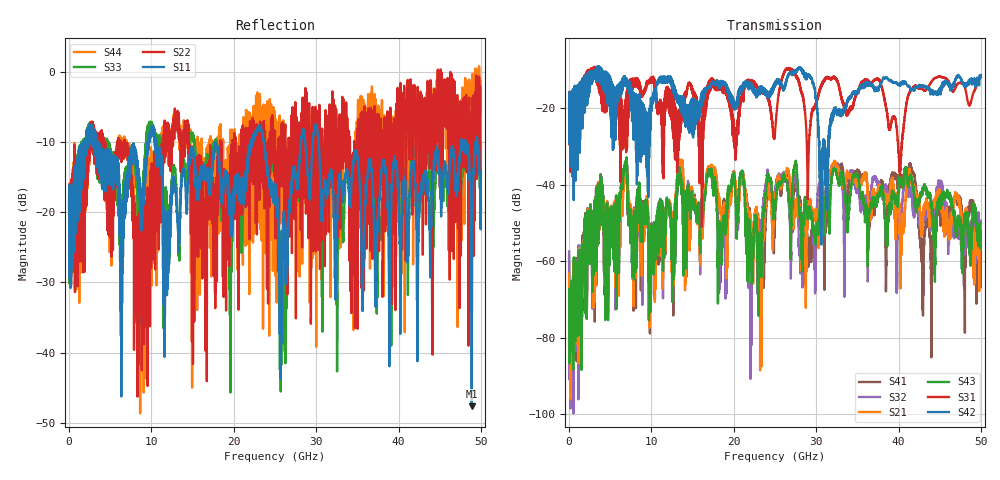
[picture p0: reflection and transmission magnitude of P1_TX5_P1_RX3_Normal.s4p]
!Keysight Technologies,N5225B,MY57041031,A.13.20.10
!Date: Friday, May 31, 2019 11:17:32
!Correction: S11(Full 4 Port(1,2,3,4))
!S12(Full 4 Port(1,2,3,4))
!S13(Full 4 Port(1,2,3,4))
!S14(Full 4 Port(1,2,3,4))
!S21(Full 4 Port(1,2,3,4))
!S22(Full 4 Port(1,2,3,4))
!S23(Full 4 Port(1,2,3,4))
!S24(Full 4 Port(1,2,3,4))
!S31(Full 4 Port(1,2,3,4))
!S32(Full 4 Port(1,2,3,4))
!S33(Full 4 Port(1,2,3,4))
!S34(Full 4 Port(1,2,3,4))
!S41(Full 4 Port(1,2,3,4))
!S42(Full 4 Port(1,2,3,4))
!S43(Full 4 Port(1,2,3,4))
!S44(Full 4 Port(1,2,3,4))
!S4P File: Measurements: <S11,S12,S13,S14>,
!<S21,S22,S23,S24>,
!<S31,S32,S33,S34>,
!<S41,S42,S43,S44>:
# Hz S  dB  R 50.0
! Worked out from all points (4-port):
!   5000 points, 10 MHz to 50 GHz, reference 50 ohm
!   strongest paths, dB at 10 MHz, 12.51 GHz, 25.01 GHz, 37.51 GHz, 50 GHz:
!     S42: -19.6, -14.4, -13.6, -14.8, -11.3
!     S31: -19.4, -23.0, -26.2, -12.3, -11.7
!     S43: -82.3, -55.2, -46.9, -42.6, -52.2
!     S21: -63.2, -53.7, -44.7, -41.9, -55.9
!     S32: -57.4, -53.5, -41.6, -39.7, -49.3
!     S41: -58.7, -54.5, -49.3, -42.6, -57.3
!   lowest |S11| = -47.7 dB at 48.9 GHz (marker M1), VSWR 1.01, Z = 49.6 + j0.00472 ohm
!   |S11| at or under -10 dB: 3.502 GHz to 9.556 GHz (6.054 GHz wide, 92.7 % of centre); 10.5 GHz to 22.11 GHz (11.6 GHz wide, 71.2 % of centre); 30.29 GHz to 47.6 GHz (17.31 GHz wide, 44.4 % of centre)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
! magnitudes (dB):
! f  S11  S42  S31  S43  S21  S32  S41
! 10 MHz  -19.7  -19.6  -19.4  -82.3  -63.2  -57.4  -58.7
! 6.81 GHz  -17.0  -12.7  -21.8  -34.3  -36.8  -35.4  -35.4
! 9.92 GHz  -9.0  -19.5  -12.3  -57.1  -57.2  -59.2  -56.6
! 28.07 GHz  -11.1  -9.3  -14.8  -47.1  -47.7  -53.8  -45.4
! 30.63 GHz  -19.8  -40.3  -14.0  -41.6  -42.0  -37.0  -46.1
! 48.9 GHz  -47.7  -12.9  -17.4  -52.7  -55.5  -51.9  -44.5
! 50 GHz  -18.3  -11.3  -11.7  -52.2  -55.9  -49.3  -57.3
